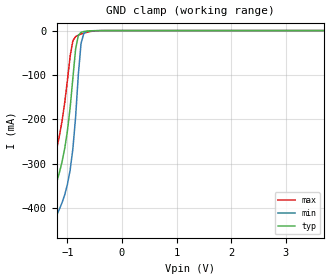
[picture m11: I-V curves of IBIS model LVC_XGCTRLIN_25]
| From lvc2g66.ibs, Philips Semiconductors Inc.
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|   Model LVC_XGCTRLIN_25
[Model]   LVC_XGCTRLIN_25
Model_type   Input
Vinl =   0.7V
Vinh =   1.7V
C_comp   3.01pF   2.23pF   3.90pF
[Model Spec]
| Note: The input and output voltage ratings may be exceeded if the input and
|   output current ratings are observed (please refer to the data sheet)
|   Subparameter   typ   min   max
| Thresholds
Vinh   1.7   1.7   1.7
Vinl   0.7   0.7   0.7
| Overshoot
S_overshoot_high   6.5   6.5   6.5   | Static overshoot
S_overshoot_low   -0.5   -0.5   -0.5
D_overshoot_high   7.2   7.2   7.2   | Dynamic overshoot
D_overshoot_low   -0.95   -0.9   -1.0
D_overshoot_time   3n   3n   3n
|Ambient temperature:   25   85   -40
[Temperature Range]   30   90   -35
[Voltage Range]   2.5V   2.3V   2.7V
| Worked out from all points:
|   GND clamp passes 1 mA (typ) near -0.61 V on its own axis
|Process Range   nominal   slow   fast
[GND_clamp]
| voltage   I(typ)   I(min)   I(max)
-5.5V     -4.553A    -4.61A     -4.497A
-1.45V    -543.2mA   -609mA     -477mA
-1.4V     -496.1mA   -562.1mA   -429.6mA
-1.35V    -449.7mA   -516.1mA   -382.9mA
-1.25V    -367.8mA   -436.8mA   -298.4mA
-1.1V     -295.9mA   -387.6mA   -204.4mA
-950mV    -173.1mA   -313.3mA   -57.16mA
-850mV    -41.37mA   -194.3mA   -13.46mA
-750mV    -3.847mA   -28.54mA   -7.836mA
-700mV    -2.146mA   -6.789mA   -5.759mA
-550mV    -554.2uA   -385.7uA   -1.497mA
5.5V      211.8pA    1.646nA    21.33pA
